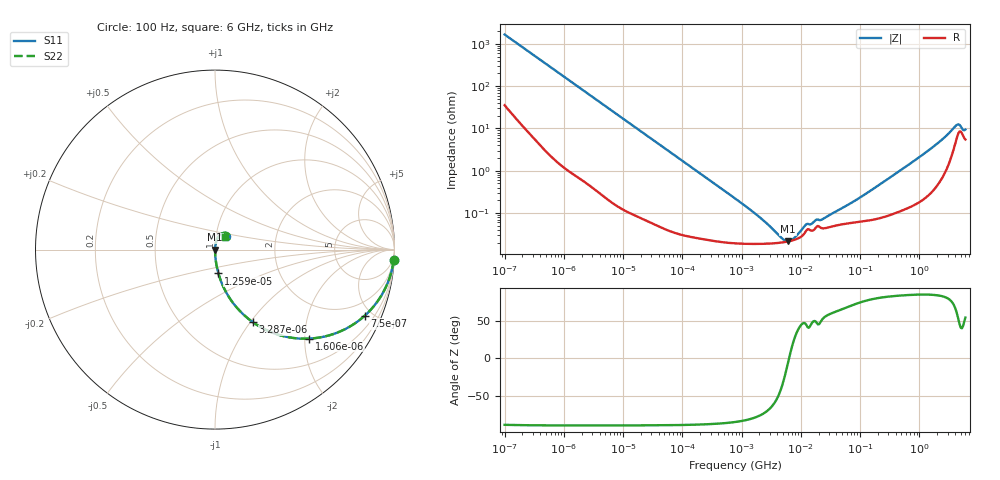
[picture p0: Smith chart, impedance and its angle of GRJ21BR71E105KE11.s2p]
!Murata Part Number: GRJ21BR71E105KE11
!These Parameters are Measured in Series Mode Connection
!Data Generated on Jun 19, 2026
!  o--ll--o
!Port1  Port2
!  o------o
!Operation Temp=25[degC], DC Bias Voltage=0[V]
!Freq. Start=100[Hz] Stop=6[GHz] 401[Steps]
# Hz S RI R 50
!Freq.(Hz) S11(Real) S11(Imag) S21(Real) S21(Imag) S12(Real) S12(Imag) S22(Real) S22(Imag)
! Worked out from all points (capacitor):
!   401 points, 100 Hz to 6 GHz, reference 50 ohm
!   read as one part in series: C = 949 nF near 109 Hz
!   lowest |Z| = 21.4 mohm at 6.075 MHz (marker M1)
!   series resonance near 6.33 MHz, so ESL is about 670 pH
!   S11 on the Smith chart (normalised r, x): 100 Hz: 2, -33; 750 Hz: 1.03, -4.50; 1.606 kHz: 1.01, -2.11; 3.287 kHz: 1.01, -1.03; 12.59 kHz: 1.00, -0.27; 6 GHz: 1.11, +0.15
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100  0.9952 -0.0594  0.00481 0.0594  0.00481 0.0594  0.9952 -0.0594
350  0.9567 -0.1985  0.0433 0.1985  0.0433 0.1985  0.9567 -0.1985
750  0.8335 -0.3689  0.1665 0.3689  0.1665 0.3689  0.8335 -0.3689
1606  0.5263 -0.4958  0.4737 0.4958  0.4737 0.4958  0.5263 -0.4958
2008  0.4165 -0.4894  0.5835 0.4894  0.5835 0.4894  0.4165 -0.4894
3287  0.2124 -0.4055  0.7876 0.4055  0.7876 0.4055  0.2124 -0.4055
5882  0.0788 -0.2661  0.9212 0.2661  0.9212 0.2661  0.0788 -0.2661
12592  0.019 -0.1328  0.981 0.1328  0.981 0.1328  0.019 -0.1328
40335  0.00228 -0.0424  0.9977 0.0424  0.9977 0.0424  0.00228 -0.0424
774597  0.000197 -0.00221  0.9998 0.00221  0.9998 0.00221  0.000197 -0.00221
2169299  0.000187 -0.000708  0.9998 0.000708  0.9998 0.000708  0.000187 -0.000708
4856642  0.000201 -0.000147  0.9998 0.000147  0.9998 0.000147  0.000201 -0.000147
6075234  0.000212 -2.24e-05  0.9998 2.24e-05  0.9998 2.24e-05  0.000212 -2.24e-05
7599586  0.00023 0.000101  0.9998 -0.000101  0.9998 -0.000101  0.00023 0.000101
1.189169e7  0.000352 0.000372  0.9996 -0.000372  0.9996 -0.000372  0.000352 0.000372
1.555665e7  0.000383 0.00042  0.9996 -0.00042  0.9996 -0.00042  0.000383 0.00042
2.327686e7  0.000436 0.000566  0.9996 -0.000566  0.9996 -0.000566  0.000436 0.000566
6.817316e7  0.000581 0.00157  0.9994 -0.00157  0.9994 -0.00157  0.000581 0.00157
3.124326e8  0.000927 0.0067  0.9991 -0.0067  0.9991 -0.0067  0.000927 0.0067
1.637704e9  0.00436 0.0346  0.9956 -0.0346  0.9956 -0.0346  0.00436 0.0346
4.193612e9  0.0597 0.0942  0.9403 -0.0942  0.9403 -0.0942  0.0597 0.0942
6e9  0.057 0.0686  0.943 -0.0686  0.943 -0.0686  0.057 0.0686
